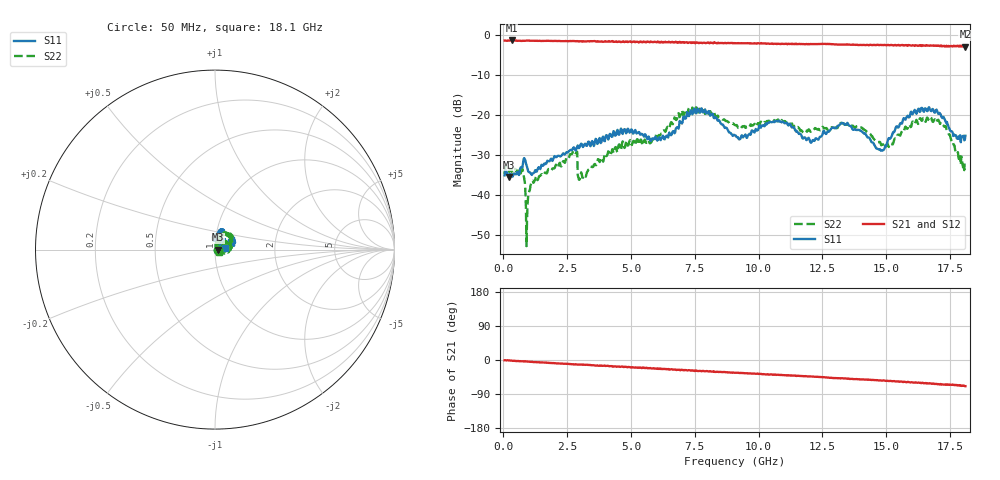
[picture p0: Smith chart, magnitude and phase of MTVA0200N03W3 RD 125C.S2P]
! Network Analyzer HP8720D.06.14 Serial No. US36140669
! 17 Jan 2005  12:17:24
! Frequency  S11  S21  S12  S22
# HZ  S  DB R 50
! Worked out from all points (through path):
!   801 points, 50 MHz to 18.1 GHz, reference 50 ohm
!   highest |S21| = -1.35 dB at 320.8 MHz (marker M1); lowest = -3.0 dB at 18.1 GHz (marker M2)
!   group delay of S21, straight-line fit = 10.1 ps
!   lowest |S11| = -35.5 dB at 207.9 MHz (marker M3), VSWR 1.03, Z = 51.7 - j0.0348 ohm
!   |S11| at or under -10 dB: start of sweep to end of sweep
!   |S22| runs from -52.9 to -18.1 dB; largest |S21 - S12| = 0.025
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5e7  -35.16 -12.4  -1.38 -0.6  -1.39 -0.8  -34.81 -4.3
2.079375e8  -35.54 -1.2  -1.37 -1.0  -1.37 -1.2  -33.96 -5.8
3.2075e8  -35.20 -0.5  -1.35 -1.6  -1.36 -1.9  -33.76 -7.2
7.494375e8  -33.10 24.4  -1.43 -3.5  -1.44 -3.6  -33.53 -12.7
9.525e8  -33.68 2.7  -1.41 -4.1  -1.38 -4.4  -42.04 46.6
1.200688e9  -34.54 26.1  -1.41 -5.6  -1.42 -5.8  -36.84 46.8
2.712375e9  -28.61 51.6  -1.49 -11.0  -1.51 -11.5  -29.46 74.8
3.073375e9  -27.34 53.8  -1.57 -12.4  -1.54 -12.8  -34.95 59.9
4.675312e9  -24.80 55.2  -1.65 -17.3  -1.69 -18.1  -26.63 70.7
6.074188e9  -26.24 63.6  -1.74 -23.7  -1.75 -23.6  -25.41 68.0
6.931562e9  -21.85 61.8  -1.87 -27.0  -1.83 -26.5  -20.24 63.1
7.563312e9  -19.62 70.8  -1.83 -28.4  -1.98 -29.7  -18.13 37.0
9.075e9  -25.13 78.3  -2.05 -33.4  -2.00 -33.8  -22.54 22.7
1.074462e10  -21.67 86.5  -2.16 -38.8  -2.17 -39.6  -21.20 20.3
1.209838e10  -26.63 71.3  -2.25 -43.8  -2.24 -44.0  -23.79 32.8
1.327162e10  -22.09 47.9  -2.38 -48.3  -2.39 -48.9  -22.02 37.3
1.476075e10  -28.66 37.3  -2.47 -53.5  -2.47 -54.0  -26.84 17.9
1.509919e10  -25.82 12.8  -2.53 -55.6  -2.46 -55.5  -28.06 30.4
1.604681e10  -19.73 18.5  -2.56 -59.2  -2.69 -59.4  -21.70 21.6
1.667856e10  -18.11 31.1  -2.69 -61.8  -2.58 -62.4  -21.38 7.6
1.728775e10  -21.10 28.7  -2.71 -64.9  -2.66 -65.2  -22.84 -12.7
1.81e10  -25.25 7.8  -2.95 -69.1  -2.86 -69.9  -31.49 -30.1
